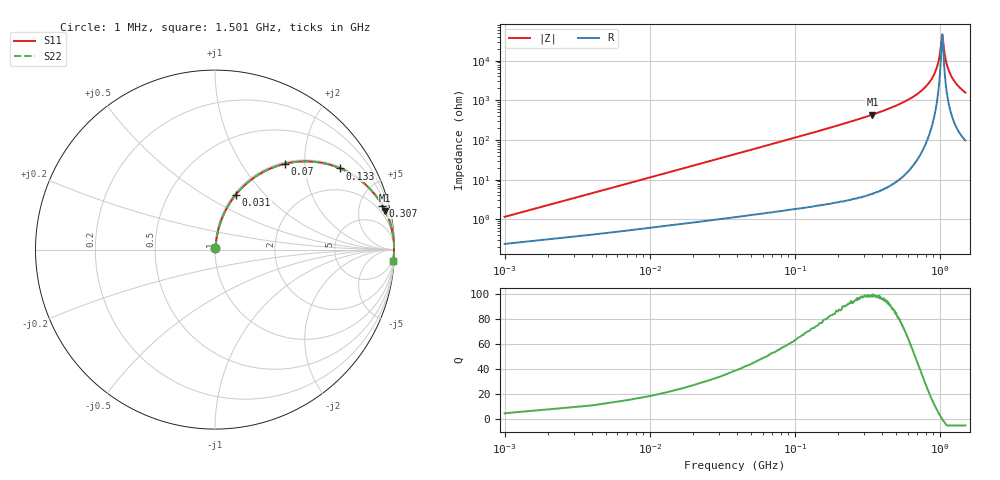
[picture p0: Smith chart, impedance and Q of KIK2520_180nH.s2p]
!version-2
!date-01.2022
!Series
# MHz S RI R 50
!Freq ReS11 ImS11 ReS21 ImS21 ReS12 ImS12 ReS22 ImS22
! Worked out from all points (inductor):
!   501 points, 1 MHz to 1.501 GHz, reference 50 ohm
!   read as one part in series: L = 180 nH near 7 MHz
!   highest Q = 98.8 at 343 MHz (marker M1), where L = 202 nH
!   self-resonance near 1.039 GHz
!   S11 on the Smith chart (normalised r, x): 1 MHz: 1.00, +0.02; 31 MHz: 1.02, +0.70; 70 MHz: 1.03, +1.59; 133 MHz: 1.04, +3.06; 307 MHz: 1.08, +7.61; 1.501 GHz: 3, -31
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1  0.00254 0.0112  0.9975 -0.0112  0.9975 -0.0112  0.00254 0.0112
10  0.0185 0.1103  0.9815 -0.1103  0.9815 -0.1103  0.0185 0.1103
13  0.0276 0.142  0.9724 -0.142  0.9724 -0.142  0.0276 0.142
22  0.0655 0.2306  0.9345 -0.2306  0.9345 -0.2306  0.0655 0.2306
31  0.1167 0.3068  0.8833 -0.3068  0.8833 -0.3068  0.1167 0.3068
70  0.3896 0.4783  0.6104 -0.4783  0.6104 -0.4783  0.3896 0.4783
133  0.698 0.4523  0.302 -0.4523  0.302 -0.4523  0.698 0.4523
253  0.8999 0.2948  0.1001 -0.2948  0.1001 -0.2948  0.8999 0.2948
307  0.9332 0.2447  0.0668 -0.2447  0.0668 -0.2447  0.9332 0.2447
343  0.9479 0.2173  0.0521 -0.2173  0.0521 -0.2173  0.9479 0.2173
502  0.9806 0.1323  0.0194 -0.1323  0.0194 -0.1323  0.9806 0.1323
751  0.9953 0.056  0.00473 -0.056  0.00473 -0.056  0.9953 0.056
916  0.9977 0.0216  0.00233 -0.0216  0.00233 -0.0216  0.9977 0.0216
967  0.9979 0.0124  0.00213 -0.0124  0.00213 -0.0124  0.9979 0.0124
1003  0.9979 0.00618  0.00211 -0.00618  0.00211 -0.00618  0.9979 0.00618
1033  0.9978 0.0012  0.00215 -0.0012  0.00215 -0.0012  0.9978 0.0012
1042  0.9978 -0.000272  0.00218 0.000272  0.00218 0.000272  0.9978 -0.000272
1078  0.9977 -0.00602  0.00232 0.00602  0.00232 0.00602  0.9977 -0.00602
1114  0.9975 -0.0116  0.00253 0.0116  0.00253 0.0116  0.9975 -0.0116
1171  0.997 -0.02  0.00299 0.02  0.00299 0.02  0.997 -0.02
1252  0.9961 -0.0314  0.00387 0.0314  0.00387 0.0314  0.9961 -0.0314
1501  0.9921 -0.0628  0.00789 0.0628  0.00789 0.0628  0.9921 -0.0628
